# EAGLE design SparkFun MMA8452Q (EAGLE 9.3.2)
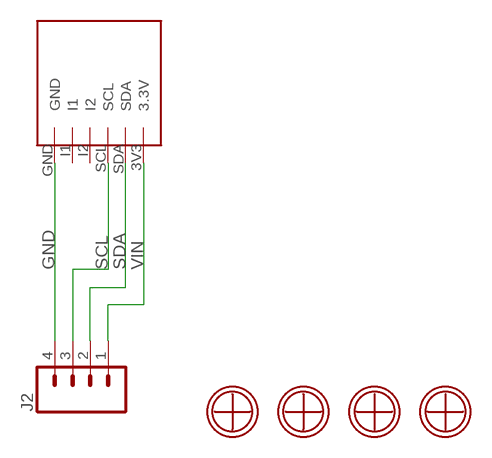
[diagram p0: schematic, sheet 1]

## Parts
J2  CONN_04  [1X04]
U$1  3.2MM-5MM  [3.2MM-5MM]
U$2  3.2MM-5MM  [3.2MM-5MM]
U$3  3.2MM-5MM  [3.2MM-5MM]
U$4  3.2MM-5MM  [3.2MM-5MM]
U$5  MMA8542Q  [MMA8542Q]

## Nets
GND: J2.4 U$5.GND
SCL: J2.3 U$5.SCL
SDA: J2.2 U$5.SDA
VIN: J2.1 U$5.3V3(3.3V)
Unconnected: U$1.P$1 U$2.P$1 U$3.P$1 U$4.P$1 U$5.I1 U$5.I2

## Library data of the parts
J2 = SparkFun-Connectors:CONN_04: Multi connection point. Often used as Generic Header-pin footprint for 0.1 inch spaced/style header connections On any of the 0.1 inch spaced packages, you can populate with these: Break Away Headers - Straight (PRT-00116) Break Away Male Headers - Right Angle (PRT-00553) Female Headers (PRT-00115)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; PROD_ID: CONN-09696
U$1-U$4 = #Holes:3.2MM-5MM
U$5 = #MMA8542Q:MMA8542Q

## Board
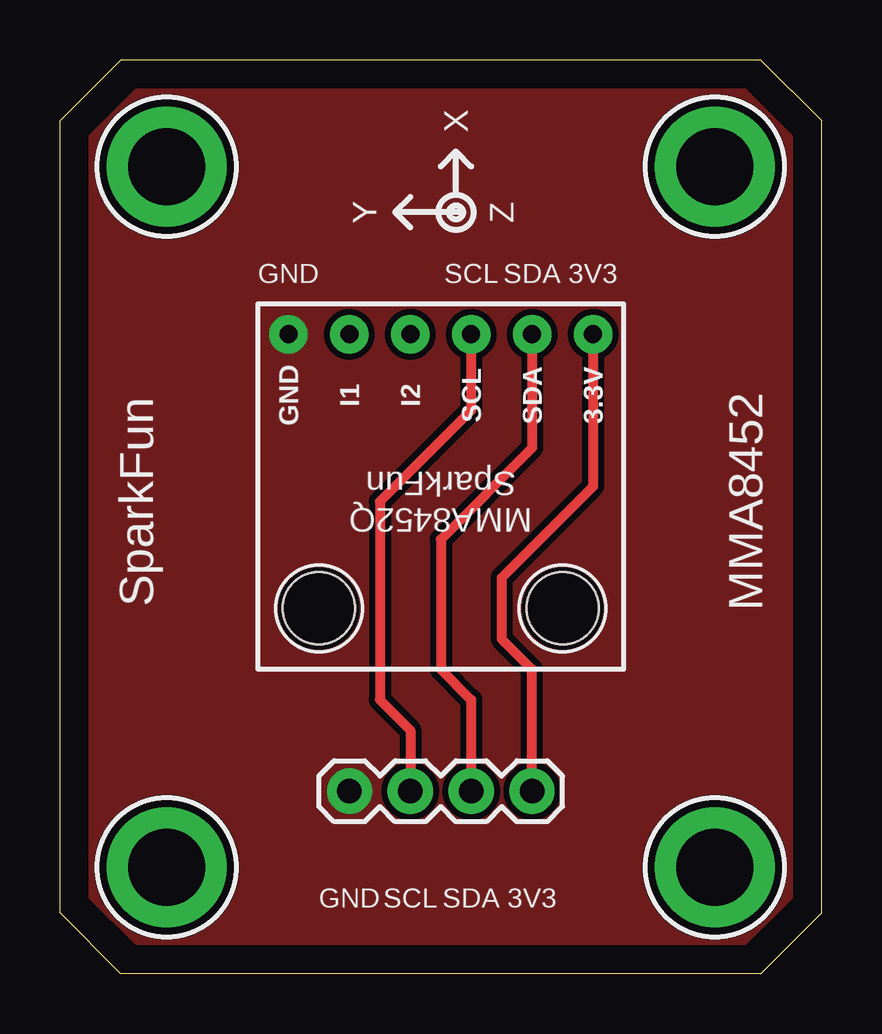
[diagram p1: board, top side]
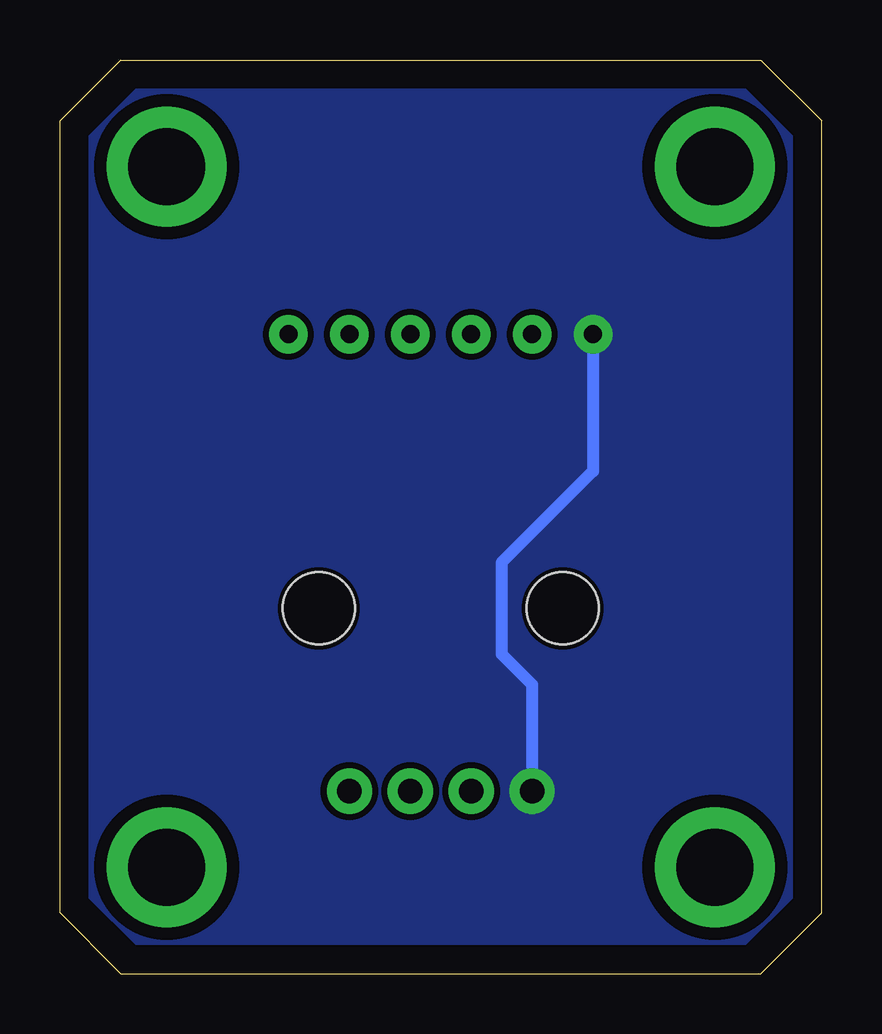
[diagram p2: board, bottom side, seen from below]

Size 31.75 x 38.1 mm. Coordinates in mm from the lower left corner, seen from the top.
Outline: 29.21,0 2.54,0 0,2.54 0,35.56 2.54,38.1 29.21,38.1 31.75,35.56 31.75,2.54 29.21,0
Copper layers (1*16): Top 0.035mm / dielectric 1.5mm / Bottom 0.035mm
Design rules "SparkFun 2 Layer Design Rule - STANDARD": minimum track width 10mil, minimum drill 20mil, track to track 10mil, track to pad 8mil, pad to pad 8mil, via to via 10mil, smd to smd 8mil, copper to edge 8mil, drill to drill 8mil, minimum pad ring 10mil, minimum via ring 10mil, stop-mask expansion 4mil, vias tented up to drill 25mil, thermal gap 10mil

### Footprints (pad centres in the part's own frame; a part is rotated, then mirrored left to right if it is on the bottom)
1X04 = drill 1.016 pad 1.88: 1 0,0; 2 2.54,0; 3 5.08,0; 4 7.62,0
3.2MM-5MM = drill 3.2 pad 5: P$1 0,0
MMA8542Q = drill 0.75 pad 1.6: 3V3 13.97,1.27; GND 13.97,13.97; I1 13.97,11.43; I2 13.97,8.89; SCL 13.97,6.35; SDA 13.97,3.81 | hole 3: 2.54,2.54; 2.54,12.7

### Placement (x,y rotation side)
J2  19.69,7.62 180 top
U$1  4.45,33.66 0 top
U$2  27.3,33.66 0 top
U$3  4.45,4.45 0 top
U$4  27.3,4.45 0 top
U$5  23.5,12.7 90 top

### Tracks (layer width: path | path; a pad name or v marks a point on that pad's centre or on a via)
GND
  Bottom 0.508: U$5.GND 9.53,20.95 13.33,17.14 13.33,13.34 12.06,12.06 J2.4
  pour Bottom (no thermals): 3.18,36.83 28.57,36.83 30.48,34.92 30.48,3.17 28.57,1.27 3.18,1.27 1.27,3.17 1.27,34.92
  pour Top (no thermals): 3.18,36.83 28.57,36.83 30.48,34.92 30.48,3.17 28.57,1.27 3.18,1.27 1.27,3.17 1.27,34.92
SCL
  Top 0.406: J2.3 14.6,10.16 13.33,11.43 13.33,19.68 17.14,23.5 U$5.SCL
SDA
  Top 0.406: U$5.SDA 19.69,21.93 15.87,18.12 15.87,12.7 17.14,11.43 J2.2
VIN
  Top 0.406: U$5.3V3 22.23,20.32 18.42,16.51 18.42,13.97 19.69,12.7 J2.1

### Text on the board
tPlace: X | Y | Z
tNames: GND | SCL | SDA | 3V3 | SparkFun | MMA8452 | GND | SCL | SDA | 3V3

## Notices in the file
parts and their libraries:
SparkFun-Connectors: Licensing: Creative Commons ShareAlike 4.0 International - https://creativecommons.org/licenses/by-sa/4.0
